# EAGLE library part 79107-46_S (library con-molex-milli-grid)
RECEPTACAL
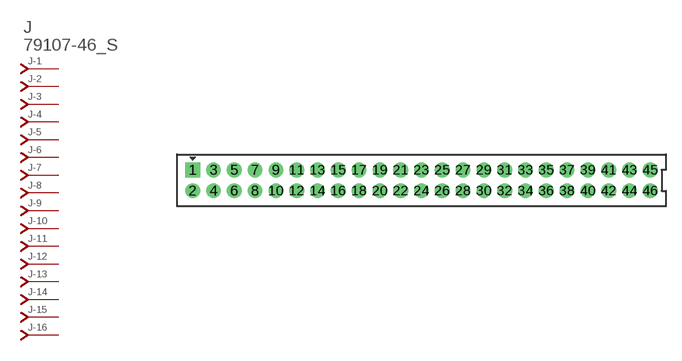
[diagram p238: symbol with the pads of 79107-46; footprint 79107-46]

Designator prefix J; gates -1=J-NV -2=J-N -3=J-N -4=J-N -5=J-N -6=J-N -7=J-N -8=J-N -9=J-N -10=J-N -11=J-N -12=J-N -13=J-N -14=J-N -15=J-N -16=J-N -17=J-N -18=J-N -19=J-N -20=J-N -21=J-N -22=J-N -23=J-N -24=J-N -25=J-N -26=J-N -27=J-N -28=J-N -29=J-N -30=J-N -31=J-N -32=J-N -33=J-N -34=J-N -35=J-N -36=J-N -37=J-N -38=J-N -39=J-N -40=J-N -41=J-N -42=J-N -43=J-N -44=J-N -45=J-N -46=J-N

## 79107-46_S  [79107-46]
1  -1:J  pas
2  -2:J  pas
3  -3:J  pas
4  -4:J  pas
5  -5:J  pas
6  -6:J  pas
7  -7:J  pas
8  -8:J  pas
9  -9:J  pas
10  -10:J  pas
11  -11:J  pas
12  -12:J  pas
13  -13:J  pas
14  -14:J  pas
15  -15:J  pas
16  -16:J  pas
17  -17:J  pas
18  -18:J  pas
19  -19:J  pas
20  -20:J  pas
21  -21:J  pas
22  -22:J  pas
23  -23:J  pas
24  -24:J  pas
25  -25:J  pas
26  -26:J  pas
27  -27:J  pas
28  -28:J  pas
29  -29:J  pas
30  -30:J  pas
31  -31:J  pas
32  -32:J  pas
33  -33:J  pas
34  -34:J  pas
35  -35:J  pas
36  -36:J  pas
37  -37:J  pas
38  -38:J  pas
39  -39:J  pas
40  -40:J  pas
41  -41:J  pas
42  -42:J  pas
43  -43:J  pas
44  -44:J  pas
45  -45:J  pas
46  -46:J  pas

## Footprint 79107-46 (pad centres in mm)
RECEPTACAL Dual Row, Vertical, Through-Hole
drill 0.914 square: 1 -22,1
drill 0.914: 2 -22,-1; 3 -20,1; 4 -20,-1; 5 -18,1; 6 -18,-1; 7 -16,1; 8 -16,-1; 9 -14,1; 10 -14,-1; 11 -12,1; 12 -12,-1; 13 -10,1; 14 -10,-1; 15 -8,1; 16 -8,-1; 17 -6,1; 18 -6,-1; 19 -4,1; 20 -4,-1; 21 -2,1; 22 -2,-1; 23 0,1; 24 0,-1; 25 2,1; 26 2,-1; 27 4,1; 28 4,-1; 29 6,1; 30 6,-1; 31 8,1; 32 8,-1; 33 10,1; 34 10,-1; 35 12,1; 36 12,-1; 37 14,1; 38 14,-1; 39 16,1; 40 16,-1; 41 18,1; 42 18,-1; 43 20,1; 44 20,-1; 45 22,1; 46 22,-1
